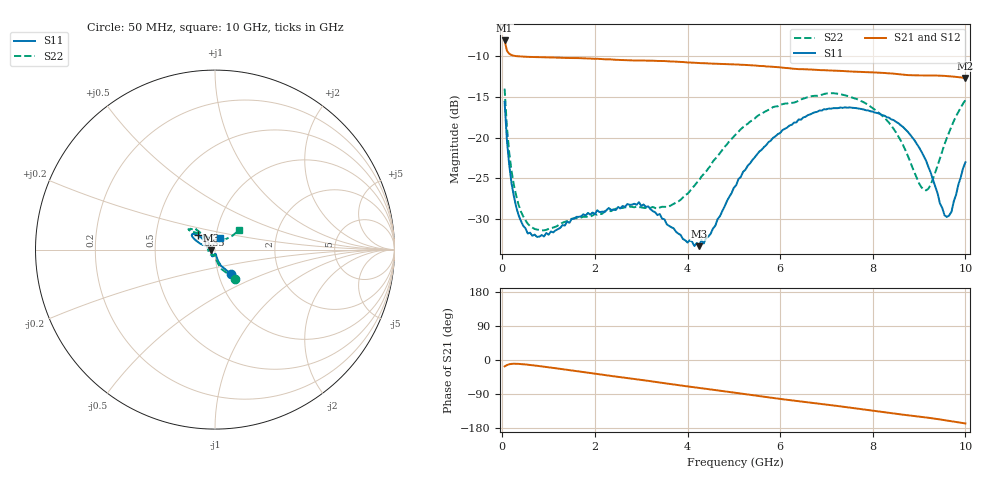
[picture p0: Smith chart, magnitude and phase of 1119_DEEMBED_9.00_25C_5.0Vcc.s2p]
!Hittite Microwave Corp.
!Digital Attenuator/PhaseShifter Rev 1.4.0
!Filename: C:\DATA\DATA\1119_DEEMBED_9.00_25C_5.0Vcc.s2p
!VNA ID: Agilent Technologies,N5224A,MY51441122,A.10.45.03
!Device type:
!2 Port Calibration.
!Temp(C): 25
!Lot Number:
!Serial Number:
!Operator:
!Misc:
!Attenuator:  9.000
# GHZ S DB R 50.0
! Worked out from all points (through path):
!   200 points, 50 MHz to 10 GHz, reference 50 ohm
!   highest |S21| = -8.11 dB at 50 MHz (marker M1); lowest = -12.7 dB at 10 GHz (marker M2)
!   group delay of S21, straight-line fit = 44.9 ps
!   lowest |S11| = -33.3 dB at 4.25 GHz (marker M3), VSWR 1.04, Z = 47.9 - j0.436 ohm
!   |S11| at or under -10 dB: start of sweep to end of sweep
!   |S22| runs from -31.4 to -14.0 dB; largest |S21 - S12| = 0.0011
!   S11 on the Smith chart (normalised r, x): 50 MHz: 1.15, -0.33; 6.35 GHz: 0.82, +0.13; 10 GHz: 1.04, +0.14
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0.05  -15.62 -56.4  -8.11 -16.9  -8.11 -16.9  -14.01 -56.0
0.1  -20.35 -69.6  -9.37 -13.4  -9.36 -13.4  -18.74 -71.2
0.15  -23.37 -74.4  -9.74 -11.2  -9.74 -11.2  -21.89 -77.7
0.25  -27.18 -77.5  -9.98 -9.9  -9.98 -9.9  -25.80 -83.8
0.4  -30.19 -79.6  -10.08 -10.7  -10.08 -10.7  -29.03 -87.5
0.55  -31.75 -80.9  -10.12 -12.4  -10.11 -12.4  -30.55 -90.4
0.9  -32.11 -87.2  -10.17 -17.6  -10.17 -17.6  -31.36 -95.9
1.75  -29.40 -104.9  -10.29 -31.7  -10.30 -31.8  -29.70 -109.2
2.95  -27.91 -111.6  -10.56 -51.7  -10.57 -51.7  -28.52 -147.0
3.4  -29.36 -122.1  -10.62 -59.3  -10.63 -59.4  -28.57 -167.4
4.25  -33.30 -167.9  -10.88 -73.7  -10.89 -73.8  -25.26 148.7
5.05  -25.84 143.8  -11.06 -86.7  -11.08 -86.8  -19.56 130.8
5.55  -21.71 139.1  -11.23 -95.2  -11.24 -95.3  -17.21 131.6
6.35  -18.15 139.5  -11.59 -107.9  -11.60 -108.0  -15.62 136.8
6.7  -17.02 141.6  -11.68 -113.1  -11.69 -113.1  -14.91 139.8
7.65  -16.40 148.8  -11.94 -127.9  -11.95 -127.9  -15.27 143.3
8.35  -17.57 152.5  -12.14 -139.3  -12.14 -139.3  -18.18 133.6
8.75  -19.26 155.6  -12.35 -145.6  -12.34 -145.6  -22.14 119.7
9.15  -22.82 158.8  -12.39 -151.6  -12.40 -151.6  -26.47 82.4
9.6  -29.72 116.7  -12.47 -159.7  -12.48 -159.7  -20.04 41.0
9.7  -29.08 94.8  -12.52 -161.6  -12.53 -161.6  -18.64 38.9
10  -23.03 68.4  -12.71 -167.4  -12.71 -167.4  -15.41 39.0
